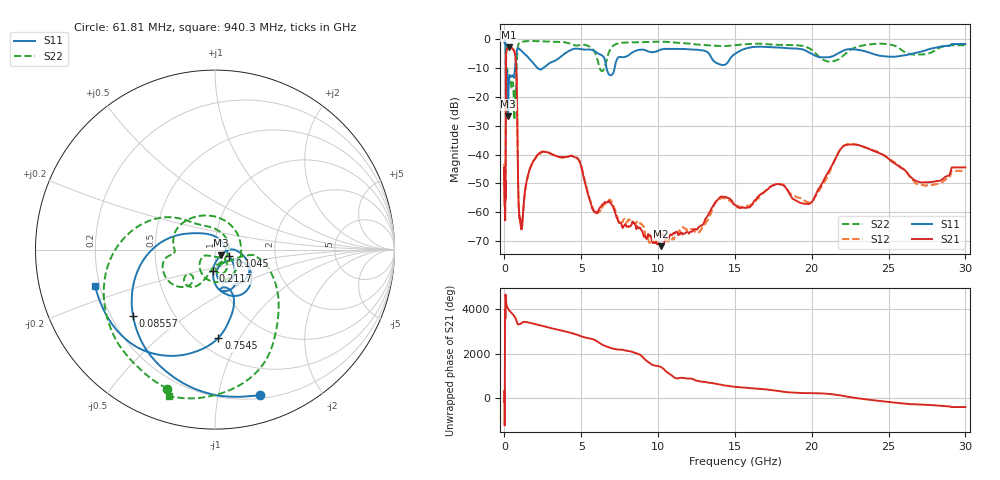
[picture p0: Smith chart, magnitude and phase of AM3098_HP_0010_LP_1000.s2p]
! Date/Time: Thu, Feb 28, 2019 8:33 AM
! Network Analyzer: Agilent Technologies E8364B Rev: A.07.50.67
! Sweep from 0.010 to 30.000 GHz, 1601 Points, Sweep Type: LOG
! Power Supply: 5.023 V, 0.002 A
# Hz S DB R 50
!freq MagS11 AngS11 MagS21 AngS21 MagS12 AngS12 MagS22 AngS22
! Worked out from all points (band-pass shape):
!   1601 points, 10 MHz to 30 GHz, reference 50 ohm
!   highest |S21| = -2.73 dB at 269.1 MHz (marker M1); lowest = -71.9 dB at 10.18 GHz (marker M2)
!   |S21| within 3 dB of the highest: 107.1 MHz to 705.9 MHz (598.8 MHz wide, 147 % of centre)
!   lowest |S11| = -26.8 dB at 235.1 MHz (marker M3), VSWR 1.10, Z = 53.4 - j3.31 ohm
!   |S11| at or under -10 dB: 92.11 MHz to 682.5 MHz (590.4 MHz wide, 152 % of centre); 2.16 GHz to 2.515 GHz (355.2 MHz wide, 15.2 % of centre); 6.644 GHz to 7.168 GHz (524 MHz wide, 7.59 % of centre)
!   |S22| runs from -28.0 to -0.5 dB; largest |S21 - S12| = 0.012
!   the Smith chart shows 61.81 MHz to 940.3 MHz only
!   S11 on the Smith chart (normalised r, x): 61.81 MHz: 0.23, -1.33; 85.57 MHz: 0.29, -0.33; 104.5 MHz: 1.17, -0.09; 211.7 MHz: 0.95, -0.23; 754.5 MHz: 0.63, -0.82; 940.3 MHz: 0.18, -0.15
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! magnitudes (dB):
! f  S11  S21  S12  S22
! 10 MHz  -0.3  -44.7  -44.9  -0.6
! 38.04 MHz  -0.5  -59.3  -60.7  -0.9
! 61.81 MHz  -1.4  -51.4  -51.5  -1.7
! 73.27 MHz  -2.1  -52.2  -54.1  -2.5
! 85.57 MHz  -4.6  -29.3  -29.3  -5.1
! 104.5 MHz  -21.0  -6.3  -6.3  -15.1
! 144.7 MHz  -15.3  -3.4  -3.4  -13.0
! 211.7 MHz  -18.4  -3.0  -2.9  -11.7
! 235.1 MHz  -26.8  -2.8  -2.8  -12.7
! 269.1 MHz  -17.3  -2.7  -2.7  -13.0
! 550.5 MHz  -12.7  -3.4  -3.4  -14.9
! 639.6 MHz  -12.7  -4.1  -4.0  -28.0
! 754.5 MHz  -6.2  -8.7  -8.7  -19.4
! 940.3 MHz  -3.1  -59.0  -59.5  -1.3
! 1.126 GHz  -4.0  -65.6  -65.5  -0.8
! 2.084 GHz  -9.6  -40.7  -40.7  -0.6
! 4.663 GHz  -3.2  -41.0  -40.9  -2.1
! 7.926 GHz  -5.9  -64.9  -63.6  -1.0
! 10.18 GHz  -3.5  -71.9  -68.6  -0.8
! 19.61 GHz  -3.9  -57.1  -56.3  -2.5
! 22.67 GHz  -3.4  -36.6  -36.4  -3.2
! 30 GHz  -1.6  -44.5  -45.7  -2.0
